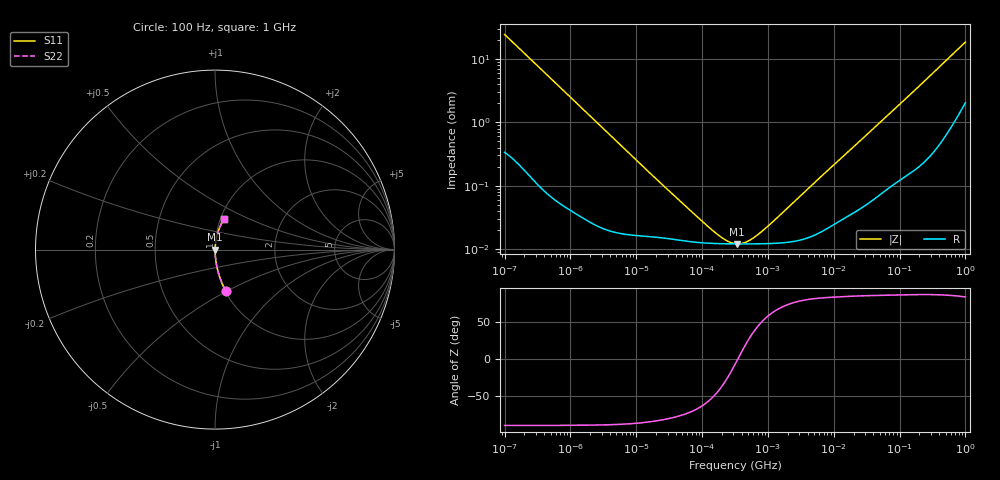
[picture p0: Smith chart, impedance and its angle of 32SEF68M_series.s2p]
!  *** S-Parameter ***
!  Copyright (C) Panasonic Industry
!  Conductive Polymer Aluminum Soild Capacitor (OS-CON)
!  Parts No. 32SEF68M
!  Connection Mode : Series
!  1  o---||---o  2
!  GND o--------o GND
!  Conditions : Temperature = 20 degC  DC Bias = 0 V
! Frequency Range : 100Hz  -  1GHz  [ 401 Steps ]
# Hz S RI R 50
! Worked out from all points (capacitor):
!   401 points, 100 Hz to 1 GHz, reference 50 ohm
!   read as one part in series: C = 64.7 uF near 108.4 Hz
!   lowest |Z| = 12 mohm at 342.8 kHz (marker M1)
!   series resonance near 348.3 kHz, so ESL is about 3.2 nH
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100  0.0595 -0.2298  0.9405 0.2298  0.9405 0.2298  0.0595 -0.2298
108.3927  0.0515 -0.2141  0.9485 0.2141  0.9485 0.2141  0.0515 -0.2141
175.7924  0.0212 -0.1372  0.9788 0.1372  0.9788 0.1372  0.0212 -0.1372
309.0295  0.00745 -0.0796  0.9925 0.0796  0.9925 0.0796  0.00745 -0.0796
613.0558  0.00221 -0.0405  0.9978 0.0405  0.9978 0.0405  0.00221 -0.0405
1487.647  0.000598 -0.0168  0.9994 0.0168  0.9994 0.0168  0.000598 -0.0168
22130.95  0.000153 -0.00115  0.9998 0.00115  0.9998 0.00115  0.000153 -0.00115
153108.7  0.000122 -0.000141  0.9999 0.000141  0.9999 0.000141  0.000122 -0.000141
229086.8  0.000121 -6.63e-05  0.9999 6.63e-05  0.9999 6.63e-05  0.000121 -6.63e-05
316227.8  0.00012 -1.49e-05  0.9999 1.49e-05  0.9999 1.49e-05  0.00012 -1.49e-05
342767.8  0.00012 -2.46e-06  0.9999 2.46e-06  0.9999 2.46e-06  0.00012 -2.46e-06
402717  0.00012 2.24e-05  0.9999 -2.24e-05  0.9999 -2.24e-05  0.00012 2.24e-05
473151.3  0.00012 4.79e-05  0.9999 -4.79e-05  0.9999 -4.79e-05  0.00012 4.79e-05
707945.8  0.00012 0.000119  0.9999 -0.000119  0.9999 -0.000119  0.00012 0.000119
1244515  0.000123 0.000253  0.9999 -0.000253  0.9999 -0.000253  0.000123 0.000253
4704354  0.00016 0.00102  0.9998 -0.00102  0.9998 -0.00102  0.00016 0.00102
6.99842e7  0.00111 0.0136  0.9989 -0.0136  0.9989 -0.0136  0.00111 0.0136
1.631173e8  0.00265 0.0307  0.9973 -0.0307  0.9973 -0.0307  0.00265 0.0307
3.235937e8  0.00693 0.06  0.9931 -0.06  0.9931 -0.06  0.00693 0.06
5.688529e8  0.0183 0.1033  0.9817 -0.1033  0.9817 -0.1033  0.0183 0.1033
9.225714e8  0.0442 0.1604  0.9558 -0.1604  0.9558 -0.1604  0.0442 0.1604
1e9  0.0511 0.1719  0.9489 -0.1719  0.9489 -0.1719  0.0511 0.1719
